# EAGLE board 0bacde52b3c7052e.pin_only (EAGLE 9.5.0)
REV: D

Size 38.1 x 22.86 mm. Coordinates in mm from the lower left corner, seen from the top.
Outline: 0,20.32 0,2.54 arc90 2.54,0 35.56,0 arc90 38.1,2.54 38.1,20.32 arc90 35.56,22.86 2.54,22.86 arc90 0,20.32
Copper layers (1*16): Top 0.035mm / dielectric 1.5mm / Bottom 0.035mm
Design rules "adafruit *": minimum track width 8mil, minimum drill 15.5mil, track to track 8mil, track to pad 8mil, pad to pad 8mil, via to via 8mil, smd to smd 8mil, copper to edge 10mil, drill to drill 8mil, minimum pad ring 10mil, minimum via ring 8mil, stop-mask expansion 2mil, vias tented up to drill 20mil, thermal gap 10mil
Net classes: 1 power: width 0.305 mm; 2 gnd: width 0.254 mm

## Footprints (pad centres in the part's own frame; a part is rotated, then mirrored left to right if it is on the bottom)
0805-NO = smd 1.24 x 1.5: 1 -0.95,0; 2 0.95,0
0603-NO = smd 1.075 x 1: 1 -0.85,0; 2 0.85,0
JST_SH4 = smd 0.6 x 1.55: 1 -1.5,2.514; 2 -0.5,2.514; 3 0.5,2.514; 4 1.5,2.514 | smd 1.2 x 1.8: MT1 -2.8,-1.386; MT2 2.8,-1.386
TP17R = smd 1.7 x 1.7: TP 0,0
_0805 = smd 1.2 x 1.3: 1 -1.016,0; 2 1.016,0
FIDUCIAL_1MM = smd 1 x 1: 1 0,0
SOT23-6 = smd 0.6 x 0.9: 1 -0.95,-1.15; 2 0,-1.15; 3 0.95,-1.15; 4 0.95,1.15; 5 0,1.15; 6 -0.95,1.15
QFN48_8MM = smd 1 x 0.23: 1 -3.9,2.75; 2 -3.9,2.25; 3 -3.9,1.75; 4 -3.9,1.25; 5 -3.9,0.75; 6 -3.9,0.25; 7 -3.9,-0.25; 8 -3.9,-0.75; 9 -3.9,-1.25; 10 -3.9,-1.75; 11 -3.9,-2.25; 12 -3.9,-2.75; 25 3.9,-2.75; 26 3.9,-2.25; 27 3.9,-1.75; 28 3.9,-1.25; 29 3.9,-0.75; 30 3.9,-0.25; 31 3.9,0.25; 32 3.9,0.75; 33 3.9,1.25; 34 3.9,1.75; 35 3.9,2.25; 36 3.9,2.75 | smd 0.23 x 1: 13 -2.75,-3.9; 14 -2.25,-3.9; 15 -1.75,-3.9; 16 -1.25,-3.9; 17 -0.75,-3.9; 18 -0.25,-3.9; 19 0.2,-3.9; 20 0.75,-3.9; 21 1.25,-3.9; 22 1.75,-3.9; 23 2.25,-3.9; 24 2.75,-3.9; 37 2.75,3.9; 38 2.25,3.9; 39 1.75,3.9; 40 1.25,3.9; 41 0.75,3.9; 42 0.25,3.9; 43 -0.25,3.9; 44 -0.75,3.9; 45 -1.25,3.9; 46 -1.75,3.9; 47 -2.25,3.9; 48 -2.75,3.9 | smd 6 x 6: THERMAL 0,0
1X11_ROUND = drill 1 pad 1.676: 1 -12.7,0; 2 -10.16,0; 3 -7.62,0; 4 -5.08,0; 5 -2.54,0; 6 0,0; 7 2.54,0; 8 5.08,0; 9 7.62,0; 10 10.16,0; 11 12.7,0
CHIPLED_0805_NOOUTLINE = smd 1.2 x 1.2: A 0,-1.05; C 0,1.05
RESONATOR-SMD = smd 0.7 x 1.7: 1 -1.2,0; 2 0,0; 3 1.2,0
EG1390 = smd 1 x 1.5: O1 -2.5,2.8; O2 -2.5,-2.8; P1 0,2.8; P2 0,-2.8; S1 2.5,2.8; S2 2.5,-2.8 | hole 1: 1.5,0; -1.5,0
SOT23-5 = smd 0.55 x 1.2: 1 -0.95,-1.3; 2 0,-1.3; 3 0.95,-1.3; 4 0.95,1.3; 5 -0.95,1.3
MOUNTINGHOLE_2.5_PLATED = drill 2.5 pad 3.2: P$1 0,0
USB_C_CUSB31-CFM2AX-01-X = smd 0.575 x 1.15: A1B12 -3.2,3.545; A4B9 -2.4,3.545; B1A12 3.2,3.545; B4A9 2.4,3.545 | smd 0.275 x 1.15: A5 -1.25,3.545; A6 -0.25,3.545; A7 0.25,3.545; A8 1.25,3.545; B5 1.75,3.545; B6 0.75,3.545; B7 -0.75,3.545; B8 -1.75,3.545 | drill 0.6 pad 1 long: M1 -4.32,2.97; M2 4.32,2.97; M3 -4.32,-1.21; M4 4.32,-1.21 | hole 0.65: 2.89,2.47; -2.89,2.47

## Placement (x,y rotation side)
C1  10uF  [0805-NO]  7.24,5.33 180 top
C2  0.1uF  [0603-NO]  23.96,17.56 90 top
C3  10uF  [0805-NO]  10.29,12.7 180 top
C4  10uF  [0805-NO]  10.79,6.6 180 top
C5  10uF  [0805-NO]  14.22,17.27 180 top
C6  0.1uF  [0603-NO]  14.48,15.75 180 top
C7  0.1uF  [0603-NO]  11.18,5.08 180 top
C8  0.1uF  [0603-NO]  22.44,17.56 90 top
C9  0.1uF  [0603-NO]  33.02,6.22 270 top
C10  10µF  [0805-NO]  31.37,6.1 270 top
CONN1  STEMMA_I2C_QT  [JST_SH4]  35.56,11.43 90 top
D+  TPTP17R  [TP17R]  3.17,9.53 0 bottom
D-  TPTP17R  [TP17R]  3.17,13.34 0 bottom
FB1  Ferrite  [_0805]  10.29,14.61 180 top
FB2  Ferrite  [_0805]  10.67,8.51 0 top
FID1  FIDUCIAL""  [FIDUCIAL_1MM]  0.97,5.26 0 top
FID2  FIDUCIAL""  [FIDUCIAL_1MM]  36.96,17.14 0 top
IC1  93LC56B  [SOT23-6]  18.54,17.51 90 top
IC2  FT232HQ  [QFN48_8MM]  17.27,10.03 0 top
JP1  [1X11_ROUND]  19.05,1.27 0 top
JP2  [1X11_ROUND]  19.05,21.59 180 top
LED1  green  [CHIPLED_0805_NOOUTLINE]  28.45,17.27 90 top
LED2  red  [CHIPLED_0805_NOOUTLINE]  32.13,17.27 90 top
Q1  12MHz  [RESONATOR-SMD]  10.67,17.27 180 top
R1  12K  [0603-NO]  25.81,17.37 90 top
R2  12K 1%  [0603-NO]  10.67,11.18 180 top
R3  1K  [0603-NO]  28.32,18.67 0 top
R4  1K  [0603-NO]  31.62,18.67 0 top
R5  2.2K  [0603-NO]  20.92,17.56 270 top
R6  5.1K  [0603-NO]  6.35,17.27 180 top
R7  12K  [0603-NO]  6.35,18.8 0 top
R8  5.1K  [0603-NO]  3.94,5.46 180 top
R9  5.1K  [0603-NO]  2.29,17.27 0 top
R10  12K  [0603-NO]  33.4,15.62 0 top
R11  12K  [0603-NO]  35.43,6.99 180 top
SW1  [EG1390]  28.19,11.43 90 top
U2  AP2112-3.3  [SOT23-5]  28.32,5.97 270 top
U$2  [ADAFRUIT_3.5MM]  22.16,3.81 0 top
U$3  [ADAFRUIT_TEXT_20MM]  31.11,11.75 0 bottom
U$4  MOUNTINGHOLE2.5  [MOUNTINGHOLE_2.5_PLATED]  2.54,20.32 0 top
U$5  MOUNTINGHOLE2.5  [MOUNTINGHOLE_2.5_PLATED]  2.54,2.54 0 top
U$6  MOUNTINGHOLE2.5  [MOUNTINGHOLE_2.5_PLATED]  35.56,20.32 0 top
U$7  MOUNTINGHOLE2.5  [MOUNTINGHOLE_2.5_PLATED]  35.56,2.54 0 top
U$8  [STEMMAQT]  35.31,7.05 90 bottom
U$11  [PCBFEAT-REV-040]  32.07,15.37 0 bottom
X6  USBC  [USB_C_CUSB31-CFM2AX-01-X]  3.17,11.43 270 top

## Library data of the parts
C1-C9 CONN1 FB1 FB2 IC2 JP1 JP2 LED1 LED2 R1-R11 SW1 U2 U$2 U$3 X6 = microbuilder
C10 = microbuilder; REV: A
D+ D- = testpad
FID1 FID2 U$4 U$5 U$7 = microbuilder; BOM: EXCLUDE
IC1 = microchip; MF: MICROCHIP; MPN: 93LC76AT-I/OT; OC_FARNELL: 1556170; OC_NEWARK: 61H6824
Q1 = SparkFun
U$6 = microbuilder; BOM: EXCLUDE; COMPANY: ADAFRUIT INDUSTRIES; DRAWN: LADYADA; REV: D
U$8 = silks
U$11 = microbuilder; REV: D

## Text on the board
tPlace: Gnd | C9 | C8 | C7 | C6 | C5 | C4 | C3 | C2 | C1 | C0 | off | I2C Mode | on | FT232H | 3V | 5V | Gnd | D0 | D1 | D2 | D3 | D4 | D5 | D6 | D7
bPlace: Gnd | C9 | C8 | C7 | C6 | C5 | C4 | C3 | C2 | C1 | C0 | FT232H | 3V logic, 5V safe | Multi-protocol USB / I2C/SPI/GPIO Chip | SCK/SCL | SDA | Connect D0 / &D1 for I2C | + | MOSI | MISO | SPICS | 3V | 5V | Gnd | D4 | D5 | D6 | D7

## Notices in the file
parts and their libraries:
microbuilder: This work is placed in the public domain, and may be freely used for commercial and non-commercial work with the following conditions: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
SparkFun: Licensing: CC v3.0 Share-Alike You are welcome to use this library for commercial purposes.
